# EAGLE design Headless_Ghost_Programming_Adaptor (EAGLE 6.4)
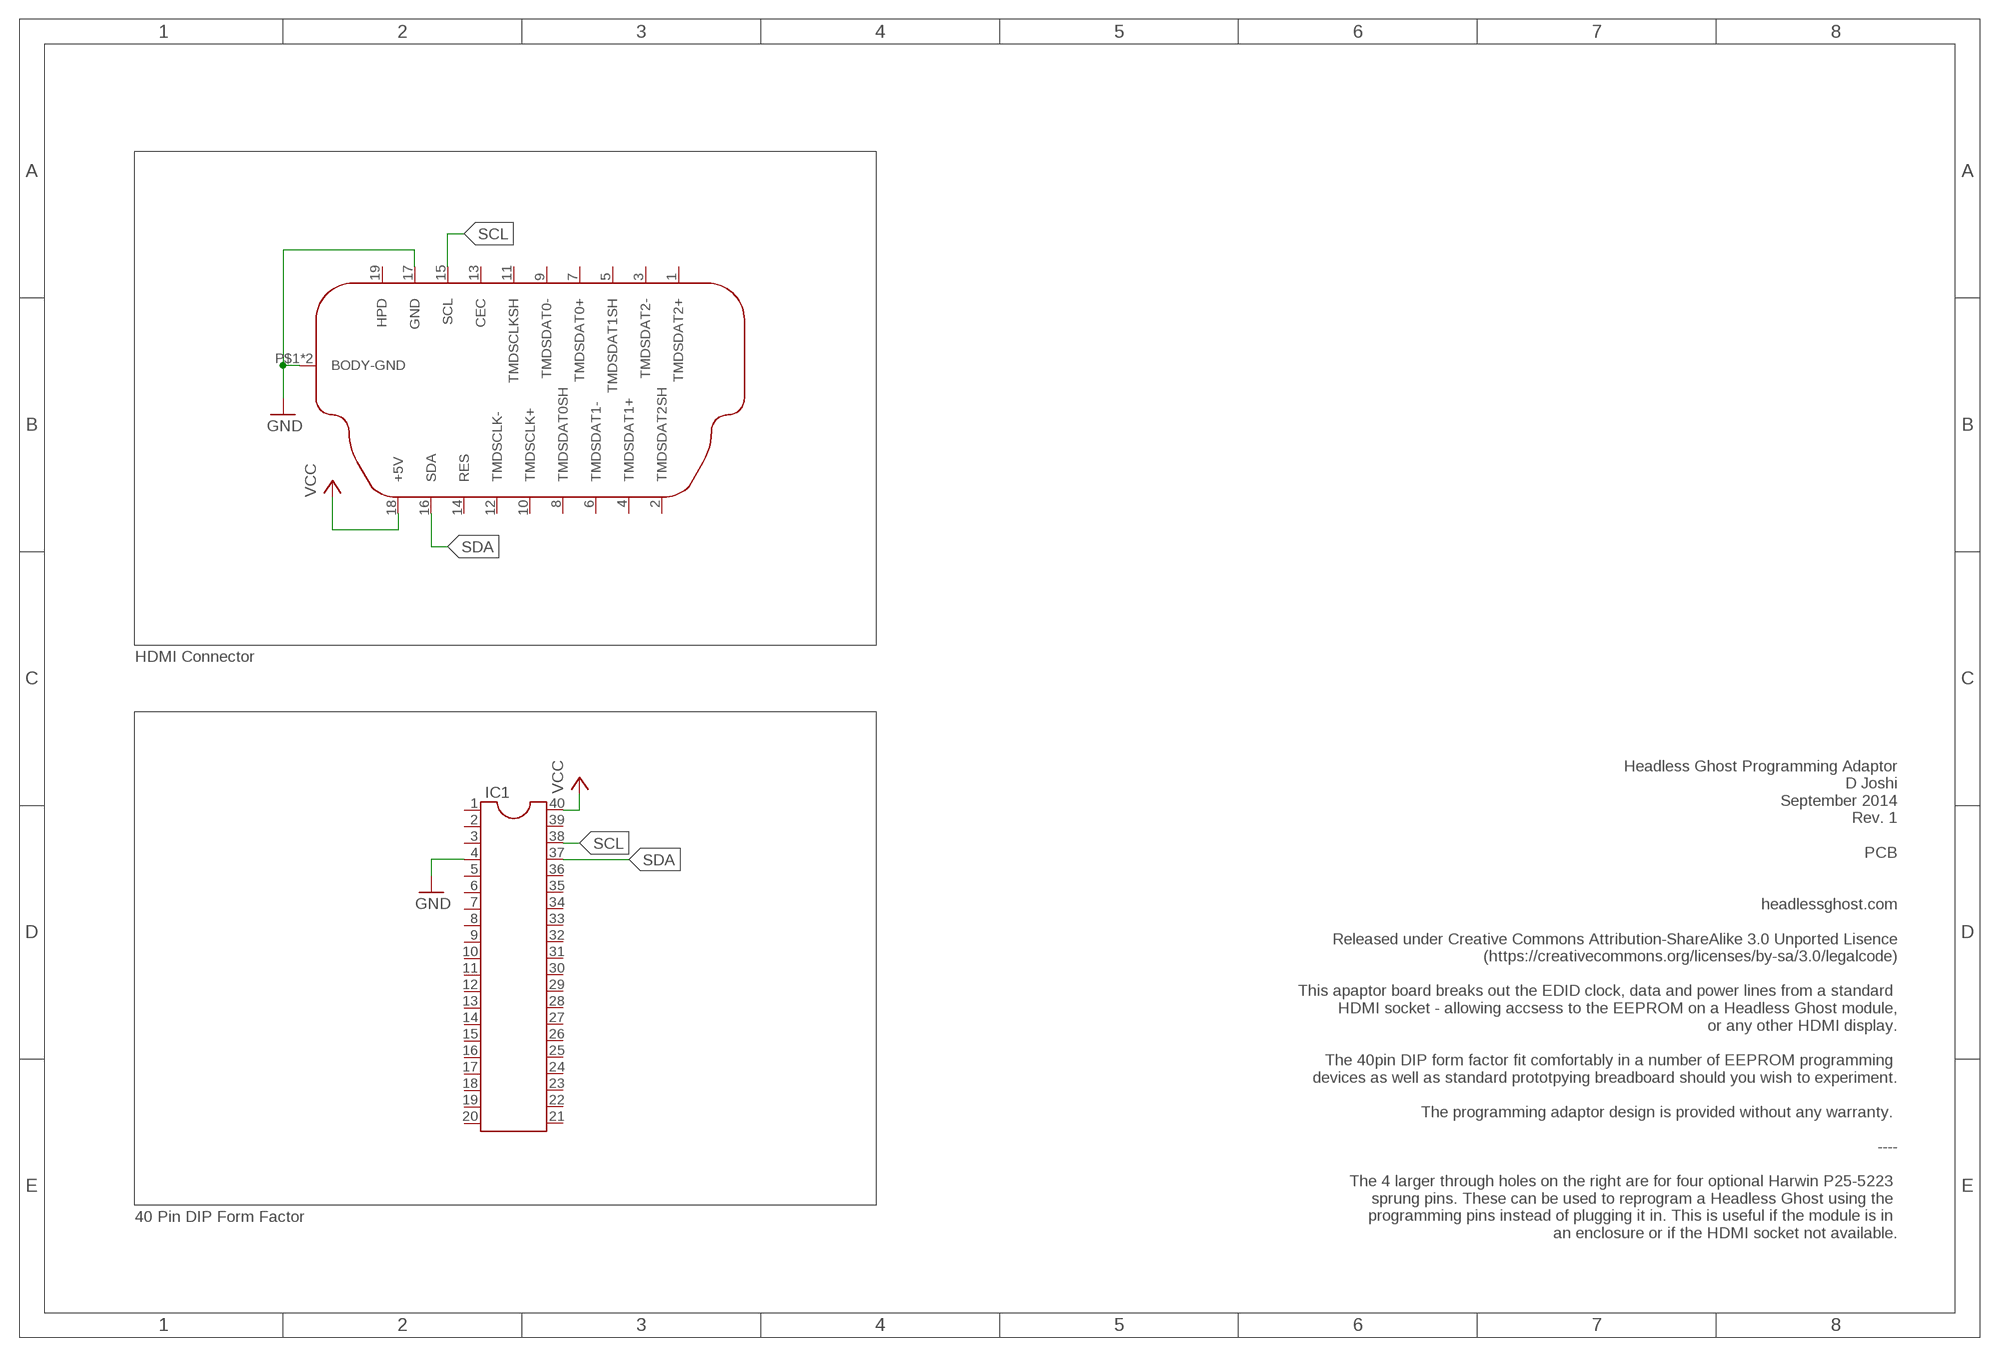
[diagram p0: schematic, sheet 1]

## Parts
IC1  DIL40  [DIL40]
U$1  HDMI-VTB-19S-GN-5  [HDMI-VTB-19S-GN-5]

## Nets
GND: IC1.4 U$1.17(GND) U$1.P$1(BODY-GND) U$1.P$2(BODY-GND)
SCL: IC1.38 U$1.15(SCL)
SDA: IC1.37 U$1.16(SDA)
VCC: IC1.40 U$1.18(+5V)
Unconnected: IC1.1 IC1.2 IC1.3 IC1.5 IC1.6 IC1.7 IC1.8 IC1.9 IC1.10 IC1.11 IC1.12 IC1.13 IC1.14 IC1.15 IC1.16 IC1.17 IC1.18 IC1.19 IC1.20 IC1.21 IC1.22 IC1.23 IC1.24 IC1.25 IC1.26 IC1.27 IC1.28 IC1.29 IC1.30 IC1.31 IC1.32 IC1.33 IC1.34 IC1.35 IC1.36 IC1.39 U$1.1(TMDSDAT2+) U$1.2(TMDSDAT2SH) U$1.3(TMDSDAT2-) U$1.4(TMDSDAT1+) U$1.5(TMDSDAT1SH) U$1.6(TMDSDAT1-) U$1.7(TMDSDAT0+) U$1.8(TMDSDAT0SH) U$1.9(TMDSDAT0-) U$1.10(TMDSCLK+) U$1.11(TMDSCLKSH) U$1.12(TMDSCLK-) U$1.13(CEC) U$1.14(RES) U$1.19(HPD)

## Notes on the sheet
- HDMI Connector
- 40 Pin DIP Form Factor
- Headless Ghost Programming Adaptor
  D Joshi
  September 2014
  Rev. 1
  
  PCB
  
  
  headlessghost.com
  
  Released under Creative Commons Attribution-ShareAlike 3.0 Unported Lisence
  (https://creativecommons.org/licenses/by-sa/3.0/legalcode)
  
  This apaptor board breaks out the EDID clock, data and power lines from a standard 
  HDMI socket - allowing accsess to the EEPROM on a Headless Ghost module,
  or any other HDMI display.
  
  The 40pin DIP form factor fit comfortably in a number of EEPROM programming 
  devices as well as standard prototpying breadboard should you wish to experiment.
  
  The programming adaptor design is provided without any warranty. 
  
  ----
  
  The 4 larger through holes on the right are for four optional Harwin P25-5223 
  sprung pins. These can be used to reprogram a Headless Ghost using the 
  programming pins instead of plugging it in. This is useful if the module is in 
  an enclosure or if the HDMI socket not available.

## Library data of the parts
IC1 = ic-package:DIL40: Dual In Line
U$1 = HDMI:HDMI-VTB-19S-GN-5: Vertical Through Hole PCB 19 pin PCB Female Connector; MANUF: TOBY; PN: HDMI-VTB-19S-GN-5

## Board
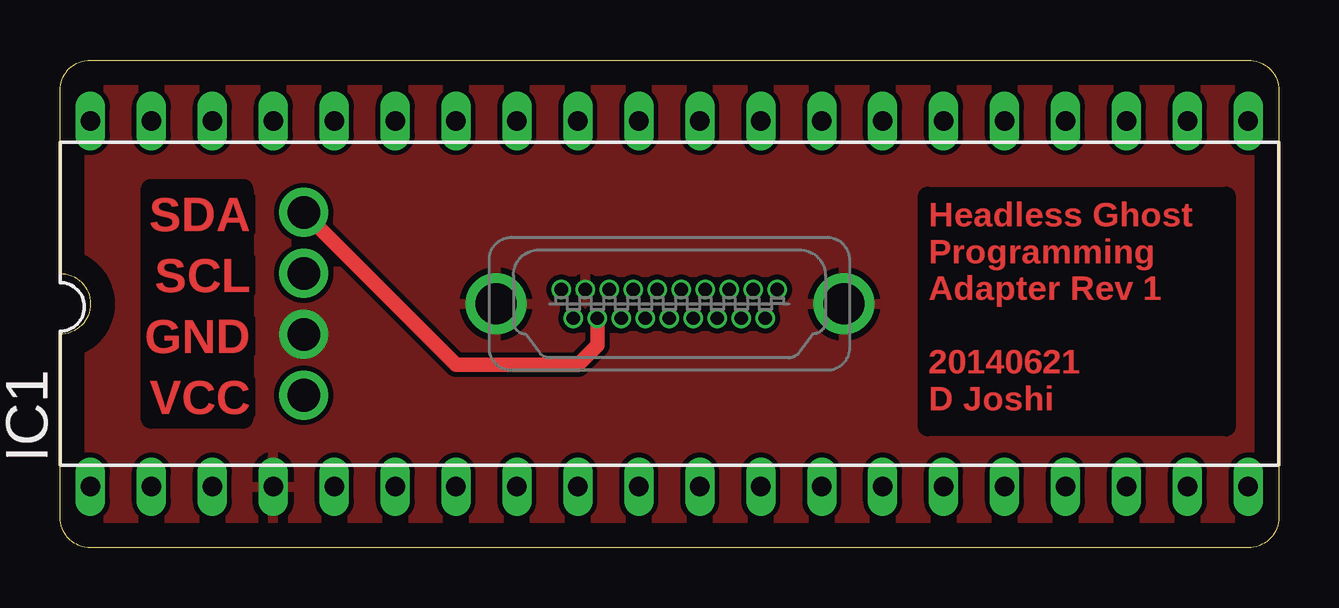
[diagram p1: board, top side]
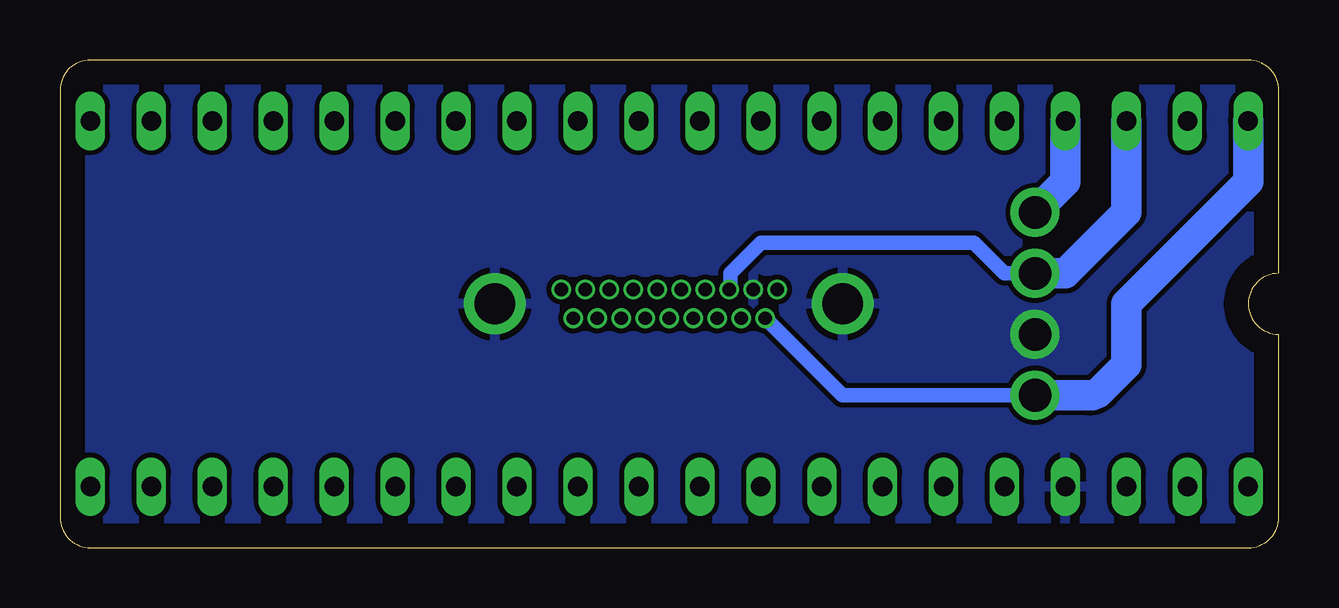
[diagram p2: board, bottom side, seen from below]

Size 50.8 x 20.32 mm. Coordinates in mm from the lower left corner, seen from the top.
Outline: 0,11.43 arc-180 0,8.89 0,1.27 arc90 1.27,0 49.53,0 arc90 50.8,1.27 50.8,19.05 arc90 49.53,20.32 1.27,20.32 arc90 0,19.05 0,11.43
Copper layers (1*16): Top 0.035mm / dielectric 1.5mm / Bottom 0.035mm
Design rules "default *": minimum track width 10mil, minimum drill 0.3mm, track to track 8mil, track to pad 8mil, pad to pad 8mil, via to via 8mil, smd to smd 8mil, copper to edge 40mil, drill to drill 8mil, minimum pad ring 1mil, minimum via ring 1mil, stop-mask expansion 4mil, vias tented up to drill 0.3mm, thermal gap 10mil
tRestrict: area 3.5,5.1 to 7.9,15.2; area 35.9,4.8 to 48.9,14.9

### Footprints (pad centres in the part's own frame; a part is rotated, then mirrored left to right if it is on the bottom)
DIL40 = drill 0.813 long: 1 -24.13,-7.62; 2 -21.59,-7.62; 3 -19.05,-7.62; 4 -16.51,-7.62; 5 -13.97,-7.62; 6 -11.43,-7.62; 7 -8.89,-7.62; 8 -6.35,-7.62; 9 -3.81,-7.62; 10 -1.27,-7.62; 11 1.27,-7.62; 12 3.81,-7.62; 13 6.35,-7.62; 14 8.89,-7.62; 15 11.43,-7.62; 16 13.97,-7.62; 17 16.51,-7.62; 18 19.05,-7.62; 19 21.59,-7.62; 20 24.13,-7.62; 21 24.13,7.62; 22 21.59,7.62; 23 19.05,7.62; 24 16.51,7.62; 25 13.97,7.62; 26 11.43,7.62; 27 8.89,7.62; 28 6.35,7.62; 29 3.81,7.62; 30 1.27,7.62; 31 -1.27,7.62; 32 -3.81,7.62; 33 -6.35,7.62; 34 -8.89,7.62; 35 -11.43,7.62; 36 -13.97,7.62; 37 -16.51,7.62; 38 -19.05,7.62; 39 -21.59,7.62; 40 -24.13,7.62
HDMI-VTB-19S-GN-5 = drill 0.55 pad 0.813: 1 4.5,0.6; 2 4,-0.6; 3 3.5,0.6; 4 3,-0.6; 5 2.5,0.6; 6 2,-0.6; 7 1.5,0.6; 8 1,-0.6; 9 0.5,0.6; 10 0,-0.6; 11 -0.5,0.6; 12 -1,-0.6; 13 -1.5,0.6; 14 -2,-0.6; 15 -2.5,0.6; 16 -3,-0.6; 17 -3.5,0.6; 18 -4,-0.6; 19 -4.5,0.6 | drill 1.7: P$1 -7.225,0; P$2 7.275,0

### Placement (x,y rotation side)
IC1  25.4,10.16 0 top
U$1  25.4,10.16 0 top

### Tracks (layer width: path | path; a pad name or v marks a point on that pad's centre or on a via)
GND  (via drill 1.36)
  other vias: 10.16,8.89
  pour Top (rank 2): -1.27,20.32 52.07,20.32 52.07,0 -1.27,0
  pour Bottom: -1.27,21.59 52.07,21.59 52.07,-1.27 -1.27,-1.27
SCL  (via drill 1.36)
  Bottom 0.61: v10.16,11.43 11.43,11.43 12.7,12.7 21.59,12.7 22.86,11.43 22.86,10.8 U$1.15
  Bottom 1.27: IC1.38 6.35,13.97 8.89,11.43 v10.16,11.43
SDA  (via drill 1.36)
  Top 0.61: v10.16,13.97 16.51,7.62 21.59,7.62 22.4,8.43 U$1.16
  Bottom 1.27: IC1.37 8.89,15.24 v10.16,13.97
VCC  (via drill 1.36)
  Bottom 0.61: v10.16,6.35 18.19,6.35 U$1.18
  Bottom 1.27: v10.16,6.35 7.88,6.35 arc-45 7.43,6.54 6.35,7.62 6.35,10.16 1.27,15.24 IC1.40

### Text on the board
Top: SDA | SCL | GND | VCC | Headless Ghost / Programming / Adapter Rev 1 / / 20140621 / D Joshi
tStop: SDA | SCL | GND | VCC | Headless Ghost / Programming / Adapter Rev 1 / / 20140621 / D Joshi
tDocu: Sprung Probes P25-5223 | Headless Ghost Programming Adaptor / D Joshi / September 2014 / Rev. 1 / / PCB / / / headlessghost.com / / Released under Creative Commons Attribution-ShareAlike 3.0 Unported Lisence / (https://creativecommons.org/licenses/by-sa/3.0/legalcode) / / This apaptor board breaks out the EDID clock, data and power lines from a standard / HDMI socket - allowing accsess to the EEPROM on a Headless Ghost module, / or any other HDMI display. / / The 40pin DIP form factor fit comfortably in a number of EEPROM programming / devices as well as standard prototpying breadboard should you wish to experiment. / / The programming adaptor design is provided without any warranty. / / ---- / / The 4 larger through holes on the right are for four optional Harwin P25-5223 / sprung pins. These can be used to reprogram a Headless Ghost using the / programming pins instead of plugging it in. This is useful if the module is in / an enclosure or if the HDMI socket not available.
